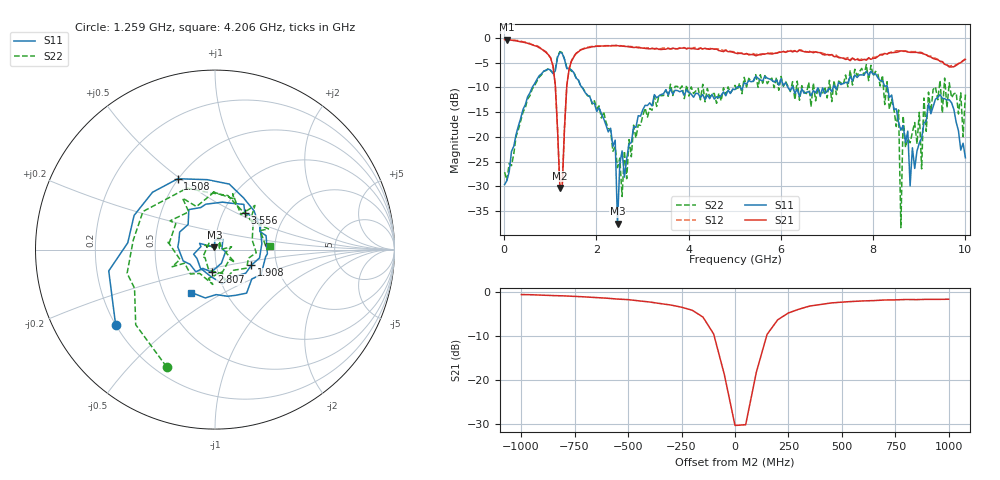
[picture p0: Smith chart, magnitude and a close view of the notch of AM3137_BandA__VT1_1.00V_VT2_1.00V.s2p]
! Date/Time: Tue, Nov 13, 2018 4:47 PM
! Network Analyzer: Agilent Technologies E8364B Rev: A.07.50.67
! Sweep from 0.010 to 10.000 GHz, 201 Points, Sweep Type: LIN
! Power Supply: 1.000 V, 0.000 A
# Hz S DB R 50
!freq MagS11 AngS11 MagS21 AngS21 MagS12 AngS12 MagS22 AngS22
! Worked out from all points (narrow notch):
!   201 points, 10 MHz to 10 GHz, reference 50 ohm
!   highest |S21| = -0.38 dB at 59.95 MHz (marker M1); lowest = -30.3 dB at 1.209 GHz (marker M2)
!   notch at M2: 27.5 dB deep, 171 MHz wide at half that depth
!   lowest |S11| = -37.6 dB at 2.458 GHz (marker M3), VSWR 1.03, Z = 49.7 + j1.28 ohm
!   |S11| at or under -10 dB: 1.686 GHz to 5.051 GHz (3.364 GHz wide, 99.9 % of centre); 6.26 GHz to 7.136 GHz (875.1 MHz wide, 13.1 % of centre); 8.309 GHz to end of sweep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
!   |S22| runs from -38.4 to -2.8 dB; largest |S21 - S12| = 0.03
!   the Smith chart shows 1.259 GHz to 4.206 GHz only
!   S11 on the Smith chart (normalised r, x): 1.259 GHz: 0.20, -0.33; 1.508 GHz: 0.50, +0.49; 1.908 GHz: 1.48, -0.27; 2.807 GHz: 0.93, -0.24; 3.556 GHz: 1.26, +0.56; 4.206 GHz: 0.69, -0.36
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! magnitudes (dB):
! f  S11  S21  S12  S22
! 10 MHz  -29.6  -0.4  -0.3  -27.1
! 59.95 MHz  -28.8  -0.4  -0.3  -28.8
! 1.009 GHz  -6.6  -4.2  -4.1  -6.7
! 1.209 GHz  -2.9  -30.3  -30.2  -2.8
! 1.259 GHz  -3.1  -30.2  -30.0  -3.0
! 1.508 GHz  -7.0  -3.9  -3.8  -6.9
! 1.708 GHz  -10.3  -2.3  -2.2  -10.2
! 1.908 GHz  -13.1  -1.8  -1.7  -13.4
! 2.408 GHz  -20.7  -1.6  -1.5  -22.0
! 2.458 GHz  -37.6  -1.6  -1.6  -26.2
! 2.807 GHz  -18.0  -2.0  -1.8  -17.7
! 3.357 GHz  -11.8  -2.3  -2.3  -11.6
! 3.556 GHz  -11.6  -2.1  -2.1  -11.8
! 4.206 GHz  -11.3  -2.3  -2.2  -10.2
! 5.005 GHz  -10.5  -3.1  -2.9  -9.6
! 6.703 GHz  -10.7  -3.0  -2.8  -9.1
! 8.352 GHz  -12.1  -3.0  -3.1  -14.5
! 8.551 GHz  -17.1  -2.8  -2.7  -14.6
! 8.601 GHz  -18.7  -2.6  -2.6  -38.4
! 8.651 GHz  -17.7  -2.7  -2.7  -15.8
! 9.051 GHz  -20.3  -3.1  -3.0  -26.5
! 10 GHz  -24.2  -4.4  -4.3  -11.5
